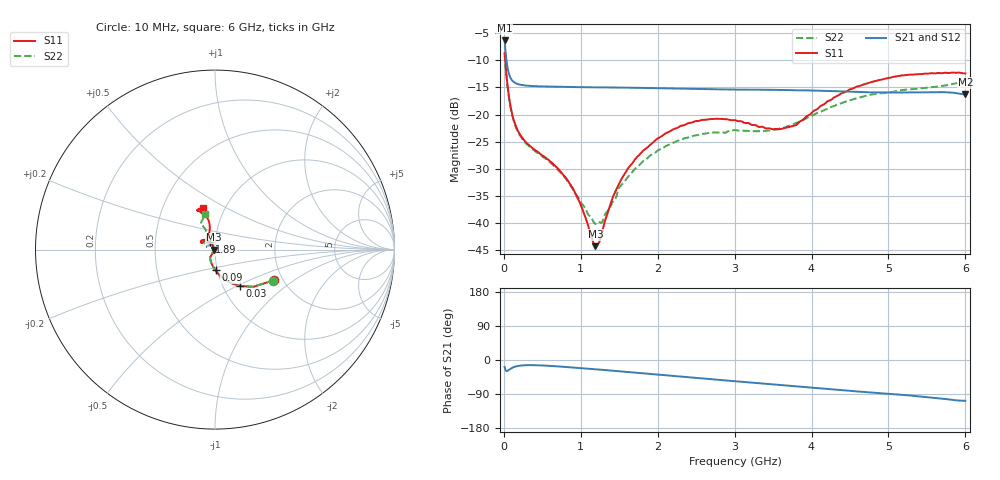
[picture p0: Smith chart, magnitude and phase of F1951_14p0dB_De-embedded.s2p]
! Integrated Device Technology
! Corporate Headquarters
! 6024 Silver Creek Valley Road
! San Jose, CA 95138  USA
! Phone:  1-408-284-8200
! Toll Free:  1-800-223-1366
! Webpage:  http://www.idt.com/
! Timing and RF Division
! 515 Groton Road, Suite 102
! Westford, MA 01886-6024
! Device:  F1951
! Description: 6-bit 0.5 dB Digital Step Attenuator
! Frequency:  100.0 -  4000.00 MHz
! Package:  4x4 mm Thin QFN Plastic Package: 24 pin
! Ports:  2 RF, 6 DC
!  Pin  1  = NC
!  Pin  2  = RF1  =  Port 1
!  Pin  3  = GND
!  Pin  4  = NC
!  Pin  5  = Serial Data Out (SDO)
!  Pin  6  = NC
!  Pin  7  = Reset Bar ( RSTb)
!  Pin  8  = Clock (CLK)
!  Pin  9  = Chip Select Bar (CSb)
!  Pin 10  = NC
!  Pin 11  = Serial Data In (SDI)
!  Pin 12  = NC
!  Pin 13  = NC
!  Pin 14  = VDD
!  Pin 15  = NC
!  Pin 16  = GND
!  Pin 17  = RF2  =  Port 2
!  Pin 18  = NC
!  Pin 19  = GND
!  Pin 20  = GND
!  Pin 21  = GND
!  Pin 22  = GND
!  Pin 23  = GND
!  Pin 24  = GND
! State:  28
! Atten State:  14.0 dB
! Voltage:  +3.30 Volts
! Current:  0.473 mA
! Data:  The device was measured on a F195X evaluation board which has
!  individual transmission lines to the RF pins.  Data was collected
!  de-embedded using a Automatic Fixture Removal [AFR] (Keysight Technologies).
!  The reference plane is the edge of the package pin.
! Misc:  Lot Code  1225BCA
!  Action Tracker AT0399
! Date Measured:  2018-09-13
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# GHz S dB R 50
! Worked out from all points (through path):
!   600 points, 10 MHz to 6 GHz, reference 50 ohm
!   highest |S21| = -6.34 dB at 10 MHz (marker M1); lowest = -16.3 dB at 6 GHz (marker M2)
!   group delay of S21, straight-line fit = 45.6 ps
!   lowest |S11| = -44.3 dB at 1.19 GHz (marker M3), VSWR 1.01, Z = 49.4 - j0.0441 ohm
!   |S11| at or under -10 dB: 17.33 MHz to end of sweep
!   |S22| runs from -40.2 to -8.7 dB; largest |S21 - S12| = 0.00037
!   S11 on the Smith chart (normalised r, x): 10 MHz: 1.80, -0.71; 30 MHz: 1.20, -0.52; 90 MHz: 0.98, -0.23; 1.89 GHz: 0.94, +0.08; 6 GHz: 0.79, +0.39
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0.01  -8.63 -27.4  -6.34 -18.3  -6.34 -18.3  -8.69 -27.9
0.03  -12.16 -55.4  -9.50 -28.8  -9.50 -28.9  -12.28 -56.1
0.09  -18.74 -88.6  -13.33 -22.8  -13.33 -22.8  -18.88 -89.8
0.16  -22.28 -105.3  -14.26 -16.9  -14.26 -16.9  -22.47 -106.5
0.25  -24.49 -115.7  -14.59 -14.1  -14.59 -14.1  -24.73 -117.6
0.72  -30.21 -120.6  -14.88 -17.1  -14.88 -17.1  -30.45 -128.0
0.88  -33.22 -120.1  -14.92 -19.5  -14.92 -19.5  -33.36 -129.4
1.01  -37.04 -123.3  -14.96 -21.5  -14.96 -21.5  -36.36 -134.2
1.19  -44.27 -175.8  -14.98 -24.4  -14.98 -24.4  -40.15 -167.9
1.28  -41.62 137.5  -14.99 -25.9  -14.99 -25.9  -39.77 165.4
1.41  -35.50 118.8  -15.02 -28.2  -15.02 -28.2  -36.19 141.9
1.53  -31.84 116.7  -15.04 -30.1  -15.04 -30.1  -32.97 133.5
1.89  -25.75 123.5  -15.12 -36.6  -15.12 -36.6  -27.70 132.3
2.01  -24.33 127.5  -15.15 -38.7  -15.15 -38.7  -26.55 134.9
2.49  -21.22 141.8  -15.27 -47.2  -15.27 -47.2  -23.86 144.7
3.01  -21.06 152.6  -15.39 -56.1  -15.40 -56.1  -22.87 149.2
3.59  -22.70 132.1  -15.46 -66.1  -15.46 -66.1  -22.54 130.9
3.79  -22.01 117.0  -15.53 -69.6  -15.53 -69.6  -21.60 123.7
4.01  -19.57 106.7  -15.57 -73.4  -15.57 -73.4  -20.20 117.9
4.49  -15.41 102.6  -15.78 -81.4  -15.78 -81.4  -17.40 116.0
5.01  -13.25 110.4  -15.95 -89.1  -15.95 -89.1  -15.99 118.5
6  -12.43 106.3  -16.30 -107.7  -16.30 -107.7  -13.74 106.0
